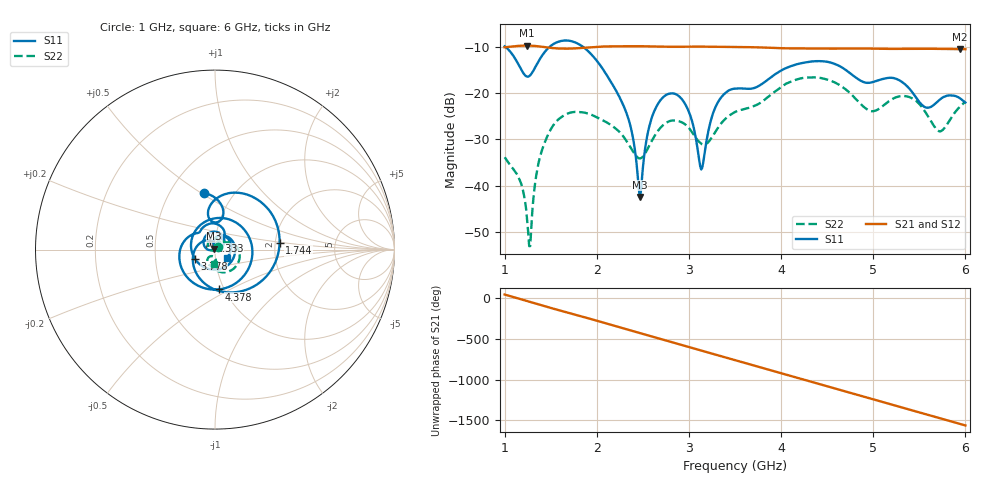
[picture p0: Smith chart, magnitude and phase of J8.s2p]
!Agilent Technologies,E8364B,MY43040528,A.07.50.67
!Agilent E8364B: A.07.50.67
!Date: Sunday, March 01, 2026 15:28:48
!Correction: S11(Full 2 Port(1,2))
!S21(Full 2 Port(1,2))
!S12(Full 2 Port(1,2))
!S22(Full 2 Port(1,2))
!S2P File: Measurements: S11, S21, S12, S22:
# Hz S  dB  R 50
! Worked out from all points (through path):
!   451 points, 1 GHz to 6 GHz, reference 50 ohm
!   highest |S21| = -9.65 dB at 1.244 GHz (marker M1); lowest = -10.4 dB at 5.944 GHz (marker M2)
!   group delay of S21, straight-line fit = 892 ps
!   lowest |S11| = -42.5 dB at 2.467 GHz (marker M3), VSWR 1.02, Z = 49.5 + j0.531 ohm
!   |S11| at or under -10 dB: 1.011 GHz to 1.485 GHz (474.2 MHz wide, 38 % of centre); 1.856 GHz to end of sweep
!   |S22| runs from -53.1 to -16.5 dB; largest |S21 - S12| = 0.0015
!   S11 on the Smith chart (normalised r, x): 1 GHz: 0.73, +0.51; 1.744 GHz: 2.11, +0.18; 2.333 GHz: 0.94, +0.10; 3.778 GHz: 0.79, -0.08; 4.378 GHz: 0.94, -0.44; 6 GHz: 1.14, -0.10
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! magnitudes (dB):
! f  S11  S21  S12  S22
! 1 GHz  -9.8  -10.0  -10.1  -33.9
! 1.167 GHz  -14.4  -9.7  -9.7  -38.9
! 1.244 GHz  -16.4  -9.7  -9.7  -47.4
! 1.278 GHz  -16.1  -9.7  -9.7  -53.1
! 1.356 GHz  -13.5  -9.8  -9.8  -36.4
! 1.456 GHz  -10.6  -10.1  -10.1  -29.7
! 1.744 GHz  -8.8  -10.3  -10.3  -24.1
! 1.844 GHz  -9.8  -10.2  -10.2  -24.1
! 2.333 GHz  -24.9  -9.8  -9.8  -30.7
! 2.467 GHz  -42.5  -9.8  -9.8  -34.1
! 2.667 GHz  -22.2  -9.9  -9.9  -28.1
! 2.933 GHz  -21.5  -9.9  -9.9  -26.4
! 3.133 GHz  -36.5  -9.9  -9.9  -30.9
! 3.289 GHz  -22.9  -9.9  -10.0  -28.3
! 3.5 GHz  -19.0  -10.0  -10.0  -24.0
! 3.778 GHz  -18.2  -10.1  -10.1  -22.0
! 4.344 GHz  -13.1  -10.3  -10.3  -16.5
! 4.378 GHz  -13.0  -10.3  -10.3  -16.5
! 5.167 GHz  -16.7  -10.4  -10.4  -21.8
! 5.722 GHz  -21.4  -10.4  -10.4  -28.3
! 5.944 GHz  -21.1  -10.4  -10.5  -22.8
! 6 GHz  -22.0  -10.4  -10.5  -21.8
